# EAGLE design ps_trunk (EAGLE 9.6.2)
DATABASE: Z:/Eigene Dateien/Anwendungsdaten/Eagle/partdb/exp.txt
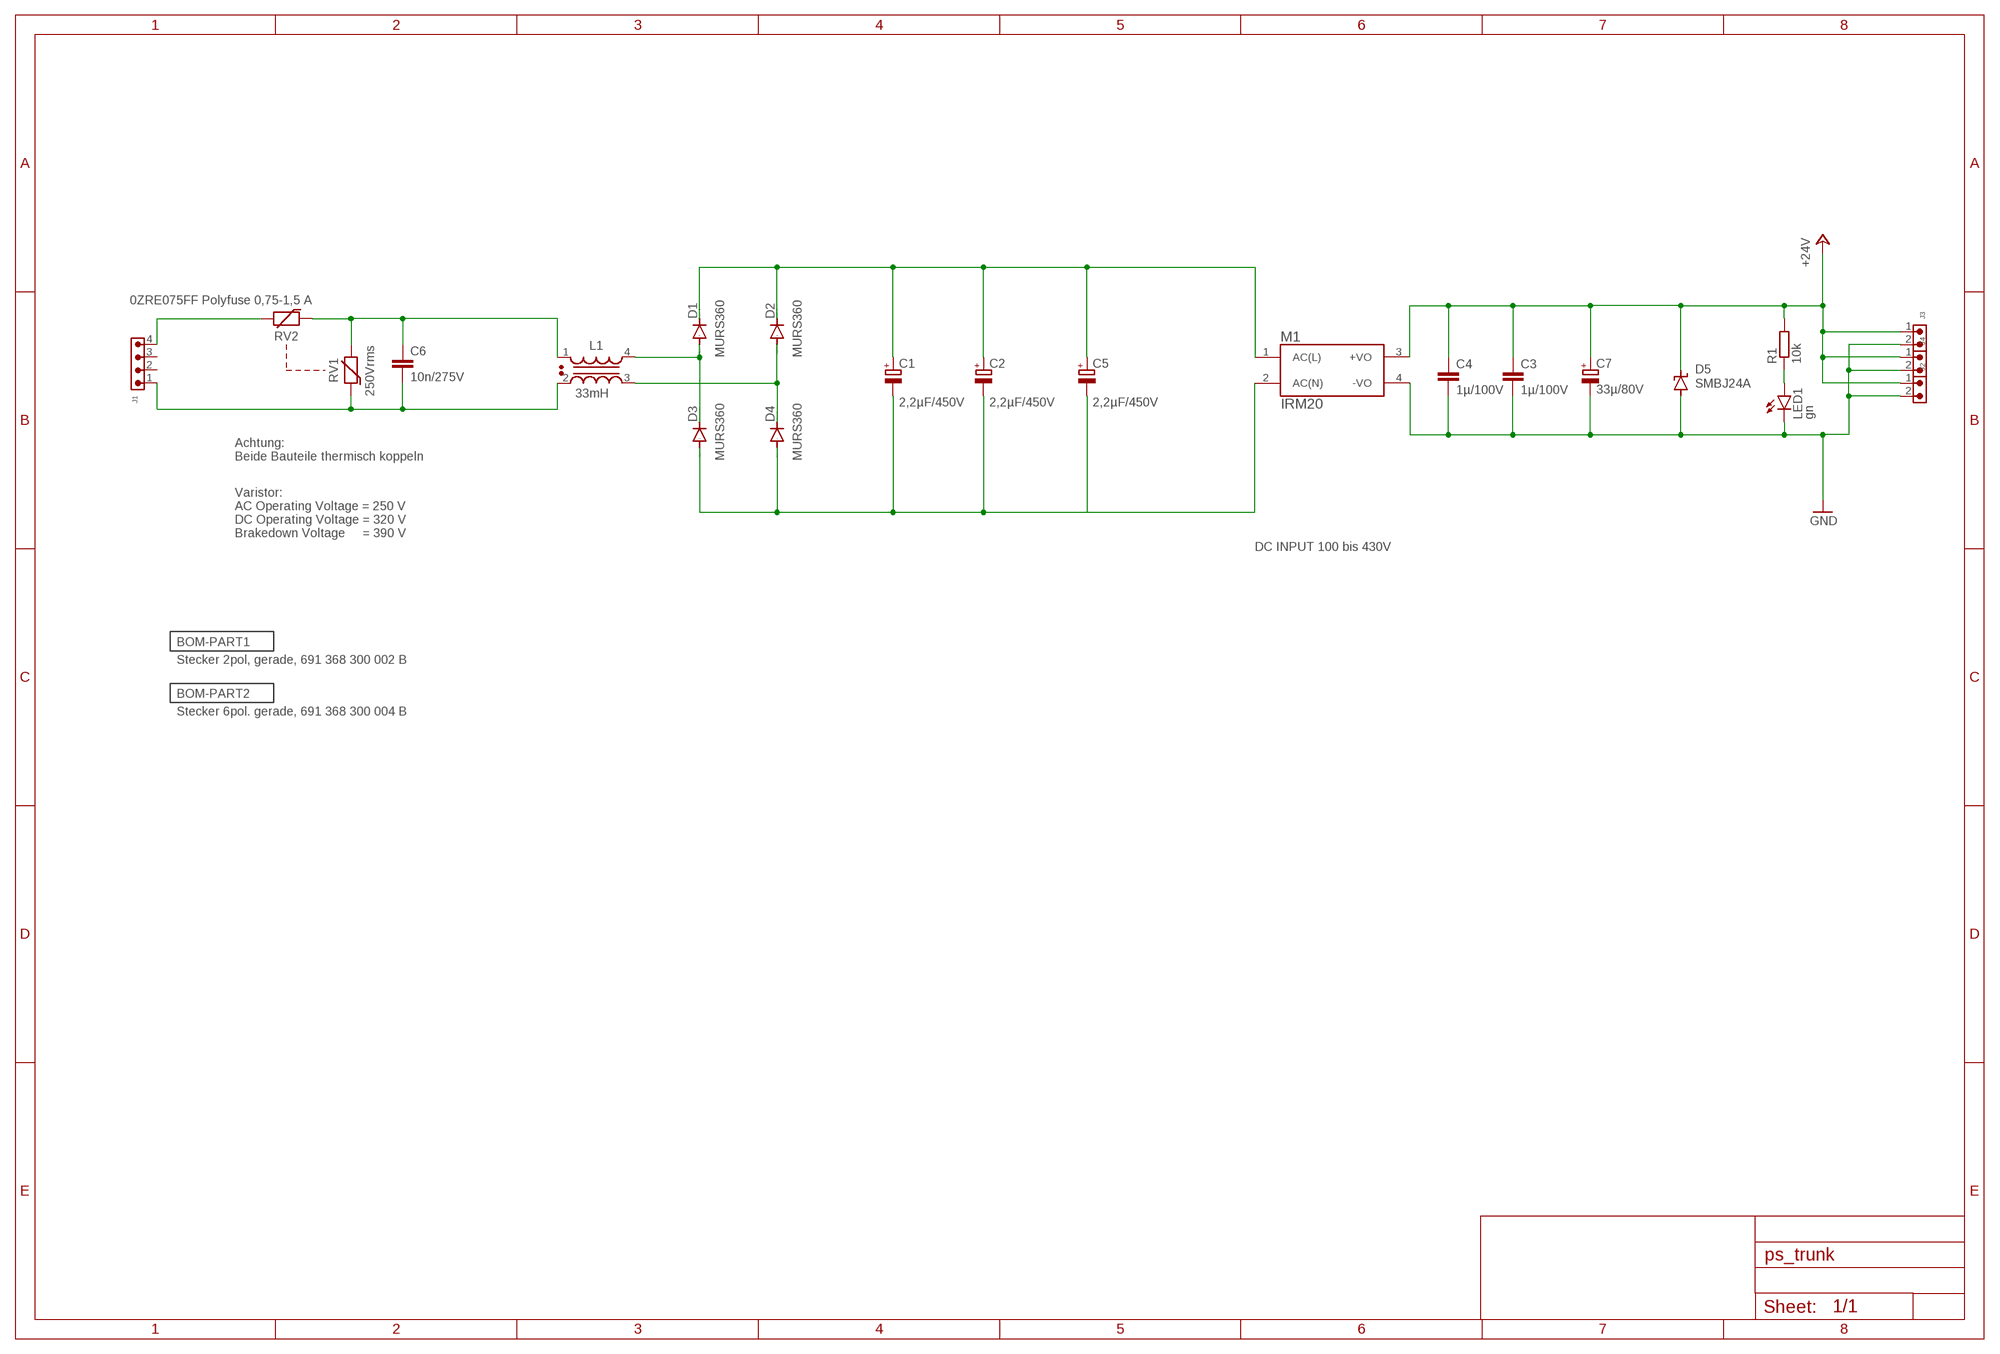
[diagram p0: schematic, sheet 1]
BOM-PART1 (BOM-PART): BOM: INCLUDE; PARTNO: CON355; QTY: 3
BOM-PART2 (BOM-PART): BOM: INCLUDE; PARTNO: CON356; QTY: 1

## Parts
C1  2,2µF/450V  CPOL-EUG  [PANASONIC_G]
C2  2,2µF/450V  CPOL-EUG  [PANASONIC_G]
C3  1µ/100V  C-EUC1210  [C1210]
C4  1µ/100V  C-EUC1210  [C1210]
C5  2,2µF/450V  CPOL-EUG  [PANASONIC_G]
C6  10n/275V  C-EU150-054X183  [C150-054X183]
C7  33µ/80V  CPOL-EUG  [PANASONIC_G]
D1  MURS360  DIODE-SMC  [SMC]
D2  MURS360  DIODE-SMC  [SMC]
D3  MURS360  DIODE-SMC  [SMC]
D4  MURS360  DIODE-SMC  [SMC]
D5  SMBJ24A  SUPPRESSOR-SMBJ  [SMBJ]
J1  691322310004  [691322310004]
J2  691322310002  [691322310002]
J3  691322310002  [691322310002]
J4  691322310002  [691322310002]
L1  33mH  WE-CMBNC_M_7448030333  [WE-CMBNC_M_7448030333]
LED1  gn  LEDCHIP-LED0603  [CHIP-LED0603]
M1  IRM20  [IRM-20]
R1  10k  R-EU_R0603  [R0603]
RV1  250Vrms  WE-VD_10MM_820512511  [WE-VD_10MM_820512511]
RV2  0ZRE075FF Polyfuse 0,75-1,5 A  WE-VD_10MM_820512511  [WE-VD_10MM_820512511]

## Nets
+24V: C3.1 C4.1 C7.+ D5.C J2.1 J3.1 J4.1 M1.3(+VO) R1.2
GND: C3.2 C4.2 C7.- D5.A J2.2 J3.2 J4.2 LED1.C M1.4(-VO)
N$1: J1.4 RV2.2
N$2: C6.2 J1.1 L1.2 RV1.1
N$3: C6.1 L1.1 RV1.2 RV2.1
N$4: LED1.A R1.1
N$5: D1.A D3.C L1.4
N$6: D2.A D4.C L1.3
N$8: C1.+ C2.+ C5.+ D1.C D2.C M1.1(AC(L))
N$9: C1.- C2.- C5.- D3.A D4.A M1.2(AC(N))
Unconnected: J1.2 J1.3

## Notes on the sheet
- Achtung:
  Beide Bauteile thermisch koppeln
- Varistor:
  AC Operating Voltage = 250 V
  DC Operating Voltage = 320 V 
  Brakedown Voltage     = 390 V
- DC INPUT 100 bis 430V

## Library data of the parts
C1 C2 C5 = rcl:CPOL-EU: POLARIZED CAPACITOR, European symbol; PARTNO: C449; SPICEPREFIX: C
C3 C4 = rcl:C-EU: CAPACITOR, European symbol; PARTNO: C216; SPICEPREFIX: C
C6 = rcl:C-EU: CAPACITOR, European symbol; PARTNO: C005; SPICEPREFIX: C
C7 = rcl:CPOL-EU: POLARIZED CAPACITOR, European symbol; PARTNO: C224; SPICEPREFIX: C
D1-D4 = diode:DIODE-: DIODE; PARTNO: D049
D5 = diode:SUPPRESSOR-: Suppressor diode; PARTNO: D212
J1 = Wurth_Connectors_WR-TBL Pluggable Connector:691322310004: WR-TBL Serie 322 - 3.81 mm Horizontal PCB Header KIND PROPERTIES Pitch 3.81 mm MATERIAL PROPERTIES Insulator Material PA66 Insulator Flammability Rating UL94 V-0 Contact Material Brass Contact Plating Tin GENERAL INFORMATION Operating Temperature -40 up to +105 °C Compliance RoHS ELECTRICAL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; DATASHEET-URL: https://www.we-online.com/catalog/datasheet/691322310004.pdf; IR-UL: 10A; IR-VDE: 10.5A; MOUNT: THT; PART-NUMBER: 691322310004; PARTNO: CON354; PINS: 4; PITCH: 3.81mm; TYPE: Horizontal; WORKING-VOLTAGE-UL: 300V (AC); WORKING-VOLTAGE-VDE: 300V (AC)
J2-J4 = Wurth_Connectors_WR-TBL Pluggable Connector:691322310002: WR-TBL Serie 322 - 3.81 mm Horizontal PCB Header; DATASHEET-URL: https://www.we-online.com/catalog/datasheet/691322310002.pdf; IR-UL: 10A; IR-VDE: 10.5A; MOUNT: THT; PART-NUMBER: 691322310002; PARTNO: CON353; PINS: 2; PITCH: 3.81mm; TYPE: Horizontal; WORKING-VOLTAGE-UL: 300V (AC); WORKING-VOLTAGE-VDE: 300V (AC)
L1 = Wurth_EMC Components_WE-CMBNC:WE-CMBNC_M: WE-CMBNC Common Mode Power Line Choke Nanocrystalline Characteristics Very high permeability nanocrystalline core material Improved isolation through plastic case and winding spacer High and stable inductance values up to 150 °C High rated currents Broadband suppression Small size Frequency range: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; DATASHEET-URL: https://www.we-online.com/catalog/datasheet/7448030333.pdf; IR: 2.5A; MOUNT: THT; PART-NUMBER: 7448030333; PARTNO: L072; RDC: 90mOhm; VR: 250 V (AC); VT: 1500 V (AC)
LED1 = led:LED: LED; PARTNO: D078
M1 = PSK-30D-24:IRM20; PARTNO: BGEK075
R1 = rcl:R-EU_: RESISTOR, European symbol; PARTNO: R221; SPICEPREFIX: R
RV1 = Wurth_EMC Components_WE-VD:WE-VD_10MM: WE-VD Disk Varistor; DATASHEET-URL: https://www.we-online.com/catalog/datasheet/820512511.pdf; ICLAMP: 25A; IPEAK: 2500A; MOUNT: THT; PART-NUMBER: 820512511; PARTNO: R055; PDISS: 0.4W; VBR: 390V; VDC: 320Vdc; WMAX: 60J
RV2 = Wurth_EMC Components_WE-VD:WE-VD_10MM: WE-VD Disk Varistor; DATASHEET-URL: https://www.we-online.com/catalog/datasheet/820512511.pdf; ICLAMP: 25A; IPEAK: 2500A; MOUNT: THT; PART-NUMBER: 820512511; PARTNO: R055; PDISS: 0.4W; VALUE: 250Vrms; VBR: 390V; VDC: 320Vdc; WMAX: 60J

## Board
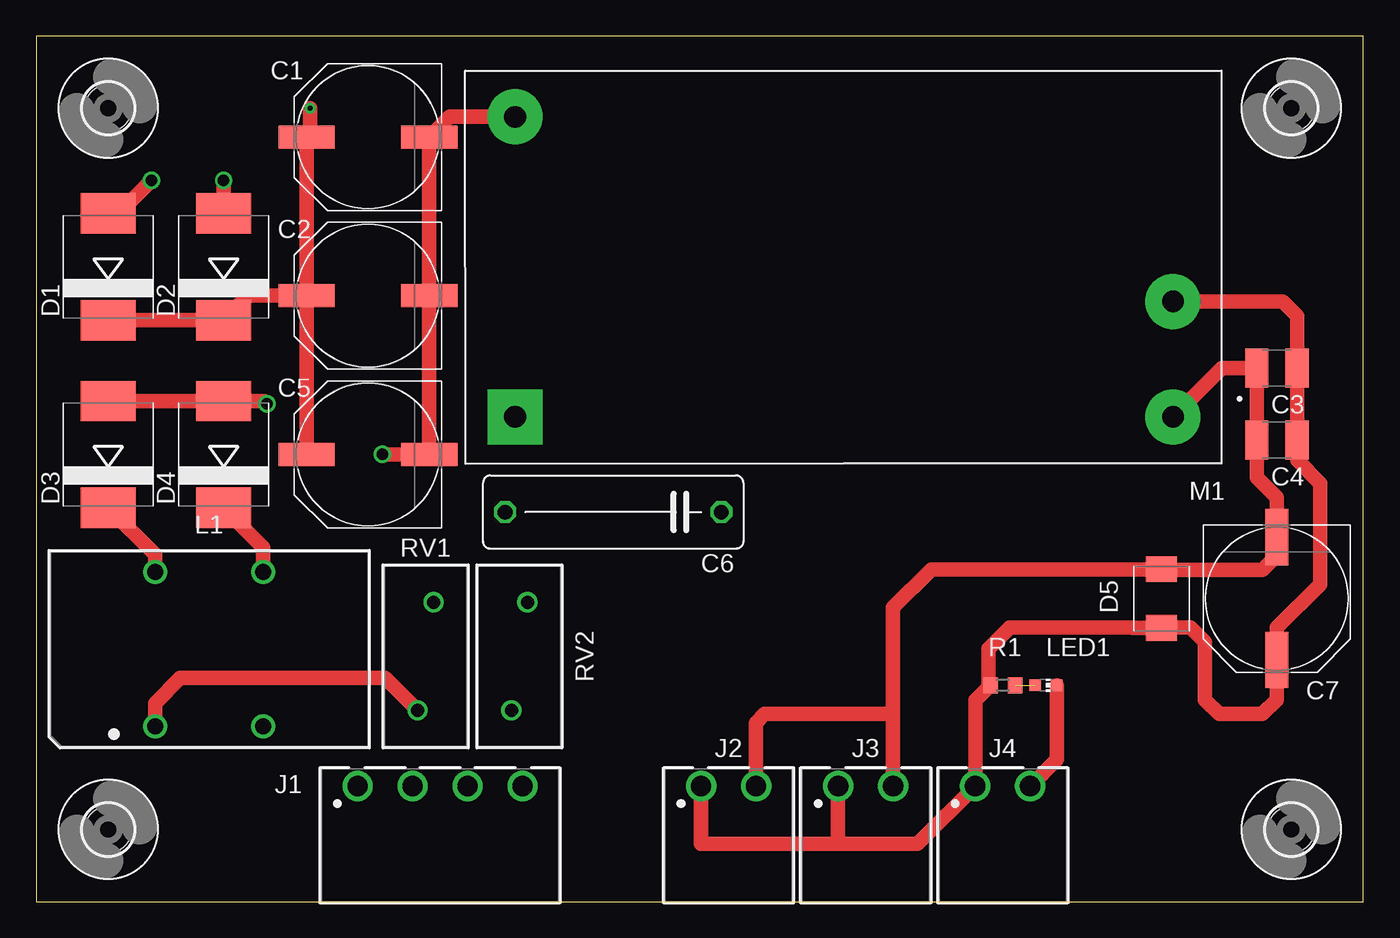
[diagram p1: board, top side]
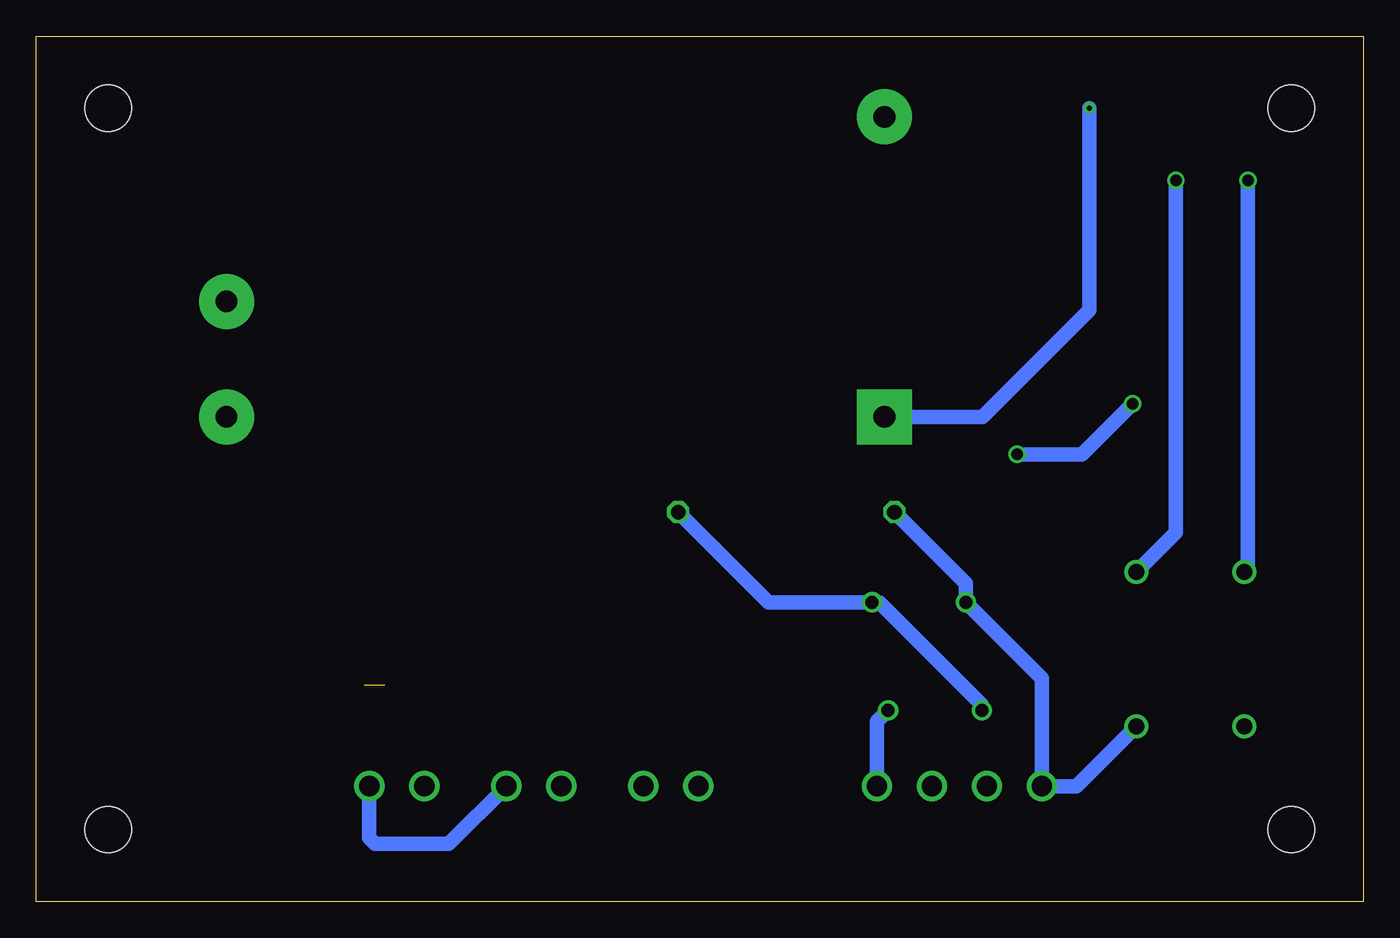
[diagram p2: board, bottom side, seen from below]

Size 92 x 60 mm. Coordinates in mm from the lower left corner, seen from the top.
Outline: 0,0 92,0 92,60 0,60 0,0
Copper layers (1*16): Top 0.035mm / dielectric 1.5mm / Bottom 0.035mm
Design rules "default": minimum track width 6mil, minimum drill 0.35mm, track to track 6mil, track to pad 6mil, pad to pad 6mil, via to via 6mil, smd to smd 6mil, copper to edge 40mil, drill to drill 6mil, minimum pad ring 10mil, minimum via ring 8mil, stop-mask expansion 4mil, vias tented up to drill 0mil, thermal gap 10mil

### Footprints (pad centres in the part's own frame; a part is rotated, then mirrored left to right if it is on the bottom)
PANASONIC_G = smd 3.9 x 1.6: + 4.25,0; - -4.25,0
C1210 = smd 1.6 x 2.7: 1 -1.4,0; 2 1.4,0
C150-054X183 = drill 1.016 octagon: 1 -7.493,0; 2 7.493,0
SMC = smd 2.8 x 3.8: A 3.7,0; C -3.7,0
SMBJ = smd 1.78 x 2.16: A 2.04,0; C -2.03,0
691322310004 = drill 1.4: 1 -5.715,0; 2 -1.905,0; 3 1.905,0; 4 5.715,0
691322310002 = drill 1.4: 1 -1.905,0; 2 1.905,0
WE-CMBNC_M_7448030333 = drill 1.1: 1 -3.75,-5.35; 2 3.75,-5.35; 3 3.75,5.35; 4 -3.75,5.35
CHIP-LED0603 = smd 0.8 x 0.8: A 0,-0.75; C 0,0.75
IRM-20 = drill 1.5 pad 3.81 square: 1 22.8,10.4 | drill 1.5 pad 3.81: 2 22.8,-10.4; 3 -22.8,2.4; 4 -22.8,10.4
R0603 = smd 1 x 1.1: 1 -0.85,0; 2 0.85,0
WE-VD_10MM_820512511 = drill 0.9: 1 -3.75,0.55; 2 3.75,-0.55
3,2 = hole 3.2: 0,0

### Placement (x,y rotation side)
C1  23,53 180 top
C2  23,42 180 top
C3  86,37 180 top
C4  86,32 180 top
C5  23,31 180 top
C6  40,27 180 top
C7  86,21 270 top
D1  5,44 90 top
D2  13,44 90 top
D3  5,31 90 top
D4  13,31 90 top
D5  78,21 90 top
J1  28,8 0 top
J2  48,8 0 top
J3  57.5,8 0 top
J4  67,8 0 top
L1  12,17.5 0 top
LED1  70,15 270 top
M1  56,44 180 top
R1  67,15 180 top
RV1  27,17 270 top
RV2  33.5,17 270 top
U$1  [3,2]  5,55 0 top
U$2  [3,2]  87,55 0 top
U$3  [3,2]  5,5 0 top
U$4  [3,2]  87,5 0 top

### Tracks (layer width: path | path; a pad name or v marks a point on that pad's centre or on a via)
+24V
  Top 0.813: R1.2 66,14.85
  Top 1.016: M1.3 86.4,41.6 87.4,40.6 C3.1 C4.1 87.4,30.6 89,29 89,22 86,19 C7.+ 86,14 85,13 82,13 81,14 81,18 80,19 78.03,19 D5.C 76.03,18.97 76,19 67.5,19 66,17.5 66,15.15 R1.2 | 66,14.85 65.09,13.95 J4.1 61.09,4 55.59,4 | J3.1 55.59,4 | J2.1 46.09,4 55.59,4
GND
  Top 1.016: M1.4 82.2,37 C3.2 C4.2 84.6,29.4 86,28 C7.- 86,24 85,23 78.04,23 D5.A 62.04,23.04 59.41,20.41 59.41,13 | LED1.C 70.75,9.85 J4.2 | J2.2 49.91,12.4 50.5,13 59.41,13 | 59.41,13 J3.2
  Bottom 1.016: J3.2 63.41,4 68.5,4 68.91,4.41 J4.2
N$1
  Bottom 1.016: J1.4 33.72,12.48 RV2.2
N$2
  Bottom 1.016: C6.2 27.55,22.04 RV1.1 22.29,15.48 J1.1 19.9,8 L1.2
N$3
  Top 1.016: L1.1 8.25,13.75 10,15.5 24.2,15.5 RV1.2
  Bottom 1.016: RV1.2 26.45,13.65 33.55,20.75 RV2.1 41.24,20.75 C6.1
N$4  (1 unrouted)
N$5  (via drill 0.8)
  Top 1.016: D3.C 8.25,24.05 L1.4 | D1.A 5.7,47.7 v8,50
  Bottom 1.016: v8,50 8,23.1 L1.4
N$6  (via drill 0.8)
  Top 1.016: L1.3 15.75,24.55 D4.C | D2.A v13,50
  Bottom 1.016: v13,50 13,25.6 L1.3
N$8  (via drill 0.35)
  Top 1.016: C5.+ C2.+ | C2.+ C1.+ 19,53.25 v19,55 | D1.C D2.C 14.7,42 C2.+
  Bottom 1.016: M1.1 26.4,33.6 19,41 v19,55
N$9  (via drill 0.8)
  Top 1.016: D3.A D4.A 15.8,34.7 v16,34.5 | M1.2 28.65,54.4 C1.- C2.- C5.- v24,31
  Bottom 1.016: v16,34.5 19.5,31 v24,31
